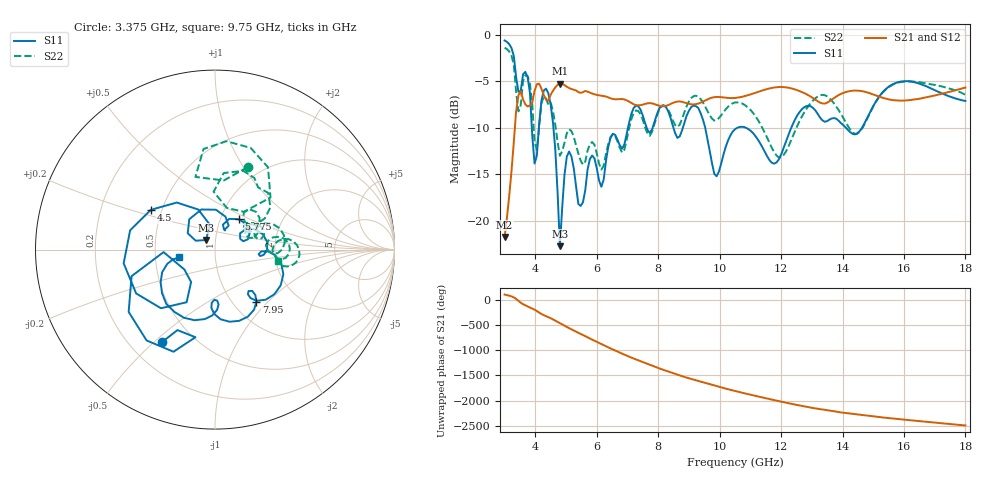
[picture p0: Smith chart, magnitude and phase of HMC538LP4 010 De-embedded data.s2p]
! Chelmsford, MA 01824
! http://www.hittite.com
! Tel: 978-250-3343
! Fax: 978-250-3373
! Device  :  HMC538LP4
! Description:  600 Analog Phase Shifter
! Frequency  :  6.0 GHz - 15.0 GHz
! Package  :  LP4  - 4x4 mm Quad Flatpack No-Lead (QFN) Plastic Package: 24 pin
! Ports  :  2 RF, 1 DC
!  Pin  3  = Rfin  = Port 1
!  Pin  16  = Rfout = Port 2
!  pin  21  = vCTL
! Voltages:  VCTL  = 0 to 5.0 Volts
! Currents :  Vb(V)  Vd(V)  Ib(mA)  Id(mA)
!  0.00  1.00  0.000000	0.484032
! Data:  The device was measured on evaluation board 111296-1.
!  Data was collected using a calibrated network analyzer.
!  The evaluation circuit board was modeled and simulated.This was use
!  to removed the evaluation board circuit from the measured data.
!  The reference plane is the center of the package pin.
! Misc:  Lot #
!Date Measured:  03 - 11 -2009
! Date:  03 - 17 -2009
! Note:
!  Hittite Microwave supplies this data as a sample of measured data at the
!  package pin for this package product.  Your particular data for this product
!  may vary.
!  Data was taken at 25 degrees C.
!  Hittite Microwave reserves the right to change this data at anytime.
# MHz S MA R 50
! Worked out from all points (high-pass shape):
!   201 points, 3 GHz to 18 GHz, reference 50 ohm
!   highest |S21| = -5.22 dB at 4.8 GHz (marker M1); lowest = -21.7 dB at 3 GHz (marker M2)
!   |S21| within 3 dB of the highest: 3.374 GHz to end of sweep
!   lowest |S11| = -22.7 dB at 4.8 GHz (marker M3), VSWR 1.16, Z = 45 + j4.85 ohm
!   |S11| at or under -10 dB: 4.59 GHz to 7.016 GHz (2.427 GHz wide, 41.8 % of centre); 9.532 GHz to 10.57 GHz (1.034 GHz wide, 10.3 % of centre); 10.87 GHz to 12.33 GHz (1.465 GHz wide, 12.6 % of centre)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
!   |S22| runs from -14.5 to -1.4 dB; largest |S21 - S12| = 0.0013
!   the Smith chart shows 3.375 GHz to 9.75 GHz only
!   S11 on the Smith chart (normalised r, x): 3.375 GHz: 0.33, -0.53; 4.5 GHz: 0.44, +0.23; 5.775 GHz: 1.22, +0.43; 7.95 GHz: 1.27, -0.86; 9.75 GHz: 0.66, -0.06
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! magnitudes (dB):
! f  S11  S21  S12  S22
! 3 GHz  -0.6  -21.7  -21.7  -1.4
! 3.375 GHz  -4.5  -8.2  -8.2  -6.1
! 3.75 GHz  -4.5  -7.7  -7.7  -4.4
! 3.975 GHz  -13.8  -6.0  -6.0  -11.5
! 4.275 GHz  -6.0  -6.5  -6.5  -6.6
! 4.5 GHz  -7.5  -6.4  -6.4  -7.3
! 4.8 GHz  -22.7  -5.2  -5.2  -13.0
! 5.1 GHz  -12.5  -5.7  -5.7  -10.1
! 5.55 GHz  -18.0  -6.2  -6.2  -14.0
! 5.775 GHz  -13.4  -6.2  -6.2  -11.8
! 6.15 GHz  -16.3  -6.5  -6.5  -14.5
! 6.525 GHz  -10.6  -6.9  -6.9  -10.7
! 7.95 GHz  -8.6  -7.5  -7.5  -8.8
! 8.025 GHz  -8.0  -7.6  -7.6  -8.1
! 9.3 GHz  -7.8  -7.4  -7.4  -6.6
! 9.75 GHz  -13.8  -6.7  -6.7  -9.0
! 10.5 GHz  -10.1  -6.8  -6.8  -7.3
! 12 GHz  -12.9  -5.6  -5.6  -13.2
! 13.05 GHz  -7.9  -6.8  -6.8  -7.0
! 14.47 GHz  -10.6  -6.0  -6.0  -10.6
! 15.53 GHz  -5.5  -6.9  -6.9  -5.6
! 18 GHz  -7.1  -5.7  -5.7  -6.4
